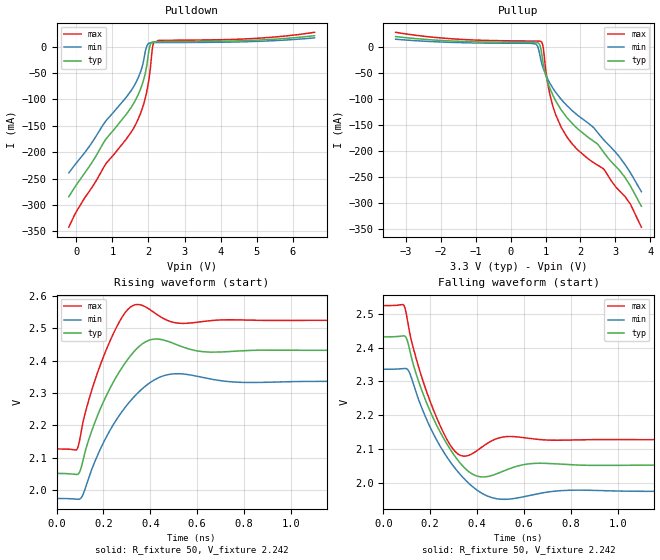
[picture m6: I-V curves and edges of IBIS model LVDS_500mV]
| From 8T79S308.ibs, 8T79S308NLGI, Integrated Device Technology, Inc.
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[Model]   LVDS_500mV
Model_type   Output
Polarity   Non-Inverting
|   typ   min   max
C_comp   2pF   1.5pF   2.5pF
Vmeas = 2.242V
Rref = 50
Cref = 0
Vref = 2.242V
|   typ   min   max
[Voltage range]   3.3V   3.135V   3.465V
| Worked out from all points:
|   slope of the pulldown table from 0 to 0.495 V, typ, clamps not added: 10.1 ohm
|   slope of the pullup table from 0 to 0.495 V, typ, clamps not added: 2.79 kohm
|   rising waveform, R_fixture 50, V_fixture 2.242: 20-80 % time 134ps typ, 160ps min, 107ps max; typ from 2.05 V to 2.43 V
|   falling waveform, R_fixture 50, V_fixture 2.242: 20-80 % time 134ps typ, 160ps min, 107ps max; typ from 2.43 V to 2.05 V
[Pulldown]
|Voltage   I (typ)   I (min)   I (max)
|Note, modeling breaks down at 250mA and above.  This is well beyond the functional   |
|operating range of the device.  Should this scenario occur, catastrophic failure and   |
|possible damage to the device and/or board is of higher concern than the I-V curve   |
|behavior.  The IBIS checker will flag currents in excess of 10A with warnings.  Lines   |
|with currents in excess of 0.35 A have been commented out.  The points still remain|
|available to the user if the user desires to use them.   |
|-1.60000e+00   -9.36160e-01   -8.30646e-01   -1.09199e+00
|-1.56720e+00   -9.10971e-01   -8.09555e-01   -1.06018e+00
|-1.55080e+00   -8.98377e-01   -7.99015e-01   -1.04427e+00
|-1.28840e+00   -6.96804e-01   -6.30512e-01   -7.89588e-01
|-1.27200e+00   -6.84198e-01   -6.19983e-01   -7.73659e-01
|-1.23920e+00   -6.58982e-01   -5.98925e-01   -7.41803e-01
|-1.22280e+00   -6.46372e-01   -5.88395e-01   -7.25878e-01
|-1.19000e+00   -6.21147e-01   -5.67334e-01   -6.94039e-01
|-1.17360e+00   -6.08534e-01   -5.56802e-01   -6.78128e-01
|-1.04240e+00   -5.07551e-01   -4.72529e-01   -5.51301e-01
|-9.76800e-01   -4.57060e-01   -4.30382e-01   -4.88336e-01
|-9.60400e-01   -4.44444e-01   -4.19845e-01   -4.73415e-01
|-9.27600e-01   -4.19229e-01   -3.98773e-01   -4.59027e-01
|-8.62000e-01   -3.73398e-01   -3.56642e-01   -4.46782e-01
|-7.96400e-01   -3.58208e-01   -3.14819e-01   -4.36622e-01
|-7.47200e-01   -3.51304e-01   -2.98376e-01   -4.29035e-01
|-4.84800e-01   -3.17875e-01   -2.67078e-01   -3.87238e-01
|-4.68400e-01   -3.15833e-01   -2.65382e-01   -3.84528e-01
-206mV    -284.4mA   -239.3mA   -342.1mA
7.2mV     -261.5mA   -220.3mA   -312mA
810.8mV   -176.3mA   -141.7mA   -223mA
1.385V    -128.3mA   -95.98mA   -175.2mA
1.713V    -91.39mA   -59.68mA   -137.9mA
1.86V     -64.09mA   -28.43mA   -110.5mA
1.959V    -33.43mA   1.599mA    -83.24mA
2.041V    1.673mA    7.07mA     -47.99mA
2.106V    8.553mA    7.564mA    -4.389mA
2.139V    9.121mA    7.615mA    7.128mA
4.73V     11.45mA    9.297mA    14.72mA
6.6V      20.66mA    16.55mA    27.05mA
[Pullup]
|Voltage   I (typ)   I (min)   I (max)
|Note, modeling breaks down at 250mA and above.  This is well beyond the functional   |
|operating range of the device.  Should this scenario occur, catastrophic failure and   |
|possible damage to the device and/or board is of higher concern than the I-V curve   |
|behavior.  The IBIS checker will flag currents in excess of 10A with warnings.  Lines   |
|with currents in excess of 0.35 A have been commented out.  The points still remain|
|available to the user if the user desires to use them.   |
-3.3V     20.66mA    15.57mA    28.83mA
719.4mV   9.373mA    6.34mA     12.05mA
818.4mV   6.56mA     -8.844mA   11.95mA
877.8mV   -7.169mA   -27.67mA   10.77mA
937.2mV   -33.15mA   -40.95mA   -2.125mA
1.016V    -56.53mA   -54.48mA   -49.19mA
1.135V    -80.51mA   -70.29mA   -93.99mA
1.452V    -120.7mA   -100.4mA   -154.2mA
1.927V    -157.1mA   -131.1mA   -197.7mA
2.68V     -203mA     -178.8mA   -234.9mA
3.432V    -266.4mA   -241mA     -301.3mA
3.749V    -305.7mA   -277.7mA   -345.9mA
| 3.90720e+00   -3.27658e-01   -3.03061e-01   -3.71247e-01
| 3.92700e+00   -3.30481e-01   -3.10958e-01   -3.74462e-01
| 3.96660e+00   -3.36159e-01   -3.35726e-01   -3.80919e-01
| 4.12500e+00   -3.60676e-01   -4.38055e-01   -4.07094e-01
| 4.16460e+00   -3.72336e-01   -4.63620e-01   -4.13706e-01
| 4.18440e+00   -3.83939e-01   -4.76399e-01   -4.17025e-01
| 4.34280e+00   -5.06400e-01   -5.78527e-01   -4.44071e-01
| 4.42200e+00   -5.67571e-01   -6.29544e-01   -4.66999e-01
| 4.50120e+00   -6.28698e-01   -6.80549e-01   -5.42262e-01
| 4.52100e+00   -6.43972e-01   -6.93301e-01   -5.61537e-01
| 4.60020e+00   -7.05036e-01   -7.44292e-01   -6.38605e-01
| 4.62000e+00   -7.20296e-01   -7.57028e-01   -6.57864e-01
| 4.65960e+00   -7.50802e-01   -7.82484e-01   -6.96373e-01
| 4.81800e+00   -8.72755e-01   -8.84423e-01   -8.50289e-01
| 4.89720e+00   -9.33731e-01   -9.36408e-01   -9.27188e-01
| 4.93680e+00   -9.64226e-01   -9.63515e-01   -9.65625e-01
| 4.95660e+00   -9.79471e-01   -9.77483e-01   -9.84838e-01
| 4.99620e+00   -1.00995e+00   -1.00622e+00   -1.02326e+00
| 5.07540e+00   -1.07081e+00   -1.06594e+00   -1.10009e+00
| 5.13480e+00   -1.11645e+00   -1.06594e+00   -1.15768e+00
| 5.45160e+00   -1.37544e+00   -1.06594e+00   -1.46512e+00
| 5.51100e+00   -1.42878e+00   -1.06594e+00   -1.52280e+00
| 5.53080e+00   -1.42878e+00   -1.06594e+00   -1.54200e+00
| 5.68920e+00   -1.42878e+00   -1.06594e+00   -1.69685e+00
| 5.76840e+00   -1.42878e+00   -1.06594e+00   -1.77900e+00
| 5.92680e+00   -1.42878e+00   -1.06594e+00   -1.95180e+00
| 5.94660e+00   -1.42878e+00   -1.06594e+00   -1.97371e+00
[Ramp]
|   typ   min   max
dV/dt_r   0.25/0.156n   0.232/0.18n   0.269/0.128n
dV/dt_f   0.25/0.156n   0.232/0.18n   0.269/0.128n
R_load =   50.0000
[Rising Waveform]
R_fixture = 50
V_fixture   =2.242  |Vcc_typ
V_fixture_min=2.155  |Vcc_min
V_fixture_max=2.326  |Vcc_max
C_fixture = 0.0p
| Time   typ   min   max
0s        2.052V     1.975V     2.127V
88.09ps   2.049V     1.972V     2.127V
136.1ps   2.153V     2.036V     2.275V
204.2ps   2.279V     2.153V     2.419V
278.3ps   2.377V     2.242V     2.532V
334.3ps   2.431V     2.291V     2.572V
410.4ps   2.466V     2.337V     2.551V
506.5ps   2.451V     2.359V     2.517V
660.7ps   2.426V     2.343V     2.523V
2ns       2.432V     2.336V     2.524V
[Falling Waveform]
R_fixture = 50
V_fixture   =2.242  |Vcc_typ
V_fixture_min=2.155  |Vcc_min
V_fixture_max=2.326  |Vcc_max
C_fixture = 0.0p
| Time   typ   min   max
0s        2.432V     2.336V     2.524V
88.09ps   2.435V     2.338V     2.524V
136.1ps   2.33V      2.274V     2.377V
204.2ps   2.204V     2.158V     2.232V
278.3ps   2.106V     2.069V     2.119V
334.3ps   2.053V     2.019V     2.08V
410.4ps   2.018V     1.973V     2.1V
506.5ps   2.033V     1.951V     2.135V
660.7ps   2.058V     1.968V     2.128V
2ns       2.052V     1.975V     2.127V
